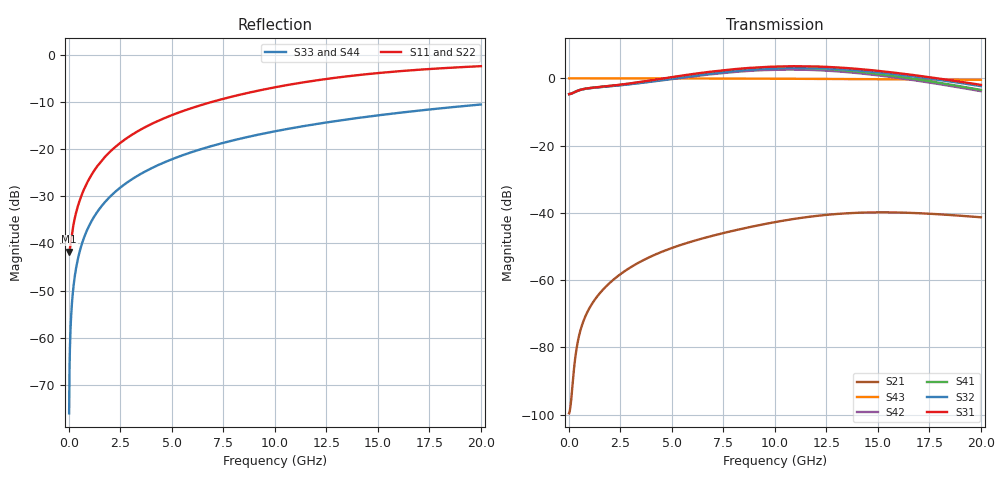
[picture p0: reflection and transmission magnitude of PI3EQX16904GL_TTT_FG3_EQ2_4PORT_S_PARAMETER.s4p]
! NPort=4 DATA=2000 NOISE=0 GROUPDELAY=0 COMPLEX_DATAFORMAT=POLAR
! NumOfBlock=1 NumOfParam=0
! .MODEL Smodel S TSTONEFILE=PI3EQX16904GL_TTT_FG3_EQ2_4PORT_S_PARAMETER.s4p TYPE=S
!  -- The above .MODEL line can be used for the S element in the netlist.
! The s parameter is extracted from the linear redriver, it is not bi-directional; only s(4,1)s(4,2) and s(3,1)s(3,2)
! should be the insertion loss
!Port definition:
!Port1 = input+
!Port2 = input-
!Port3 = output+
!Port4 = output-
# Hz S MA R  50
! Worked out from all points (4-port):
!   2000 points, 10 MHz to 20 GHz, reference 50 ohm
!   strongest paths, dB at 10 MHz, 5.01 GHz, 10.01 GHz, 15.01 GHz, 20 GHz:
!     S31: -4.7, 0.4, 3.5, 2.2, -1.9
!     S32: -4.7, -0.1, 3.0, 1.8, -2.3
!     S41: -4.7, 0.3, 3.1, 1.3, -3.4
!     S42: -4.7, -0.2, 2.6, 0.9, -3.8
!     S43: 0.0, 0.0, -0.1, -0.3, -0.4
!     S21: -99.6, -50.4, -42.7, -39.8, -41.3
!   lowest |S11| = -41.7 dB at 10 MHz (marker M1), VSWR 1.02, Z = 49.2 - j0.0603 ohm
!   |S11| at or under -10 dB: start of sweep to 6.905 GHz
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1e7  0.008182 -175.7  1.05e-05 7.6  0 0.0  0 0.0
     1.05e-05 7.6  0.008182 -175.7  0 0.0  0 0.0
     0.5834 0.2  0.5834 -179.8  0.0001571 -90.0  1 -0.0
     0.5834 -179.8  0.5834 0.2  1 -0.0  0.0001571 -90.0
3.9e8  0.02299 -119.3  0.0001042 117.2  0 0.0  0 0.0
       0.0001042 117.2  0.02299 -119.3  0 0.0  0 0.0
       0.6474 4.9  0.6465 -175.5  0.006126 -90.4  1 -0.4
       0.6474 -175.8  0.6464 3.8  1 -0.4  0.006126 -90.4
1.65e9  0.07835 -102.7  0.0007211 104.2  0 0.0  0 0.0
        0.0007212 104.2  0.07835 -102.7  0 0.0  0 0.0
        0.753 -3.6  0.7465 175.1  0.02591 -91.5  0.9996 -1.5
        0.752 173.4  0.7455 -7.9  0.9996 -1.5  0.02591 -91.5
6.1e9  0.2798 -105.4  0.003878 74.4  0 0.0  0 0.0
       0.003864 74.3  0.2798 -105.5  0 0.0  0 0.0
       1.168 -43.0  1.097 135.8  0.09535 -95.7  0.9951 -5.5
       1.147 126.2  1.077 -55.1  0.9951 -5.5  0.09535 -95.7
9.98e9  0.4535 -113.0  0.007325 45.4  0 0.0  0 0.0
        0.00727 45.7  0.4526 -113.1  0 0.0  0 0.0
        1.496 -99.9  1.407 80.3  0.1547 -99.3  0.987 -8.9
        1.425 62.7  1.341 -117.1  0.987 -8.9  0.1547 -99.3
1.411e10  0.6149 -123.0  0.0101 6.1  0 0.0  0 0.0
          0.01007 6.6  0.6132 -123.0  0 0.0  0 0.0
          1.374 -167.1  1.303 13.6  0.216 -103.0  0.9745 -12.5
          1.252 -10.9  1.188 169.8  0.9745 -12.5  0.216 -103.0
2e10  0.762 -135.6  0.008672 -38.4  0 0.0  0 0.0
      0.008608 -38.0  0.7607 -135.5  0 0.0  0 0.0
      0.7995 110.7  0.7653 -68.4  0.2986 -108.1  0.9506 -17.4
      0.6731 -101.3  0.6444 79.6  0.9506 -17.4  0.2986 -108.1
